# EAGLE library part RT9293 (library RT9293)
USB Filter with ESD Protection Source: http://www.onsemi.com/pub_link/Collateral/NUF2101M-D.PDF
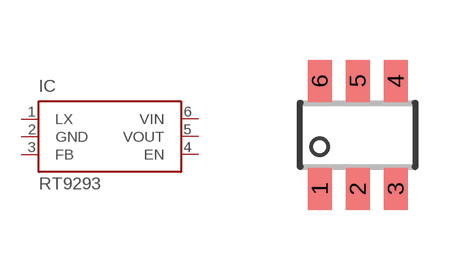
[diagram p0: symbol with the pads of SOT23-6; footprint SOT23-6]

Designator prefix IC

## RT9293 (MF: ON Semiconductor; MPN: NUF2101MT1; OC_FARNELL: unknown; OC_NEWARK: unknown), RT9293G (MF: ON Semiconductor; MPN: NUF2101MT1G; OC_FARNELL: unknown; OC_NEWARK: 04R7860)  [SOT23-6]
1  LX  pas
2  GND  pas
3  FB  pas
4  EN  pas
5  VOUT  pas
6  VIN  pas

## Footprint SOT23-6 (pad centres in mm)
SOT-23-6 (TSOP-6) Plastic Small Outline - 6-Lead Package
smd 0.6 x 1.05: 1 -0.95,-1.35; 2 0,-1.35; 3 0.95,-1.35; 4 0.95,1.35; 5 0,1.35; 6 -0.95,1.35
